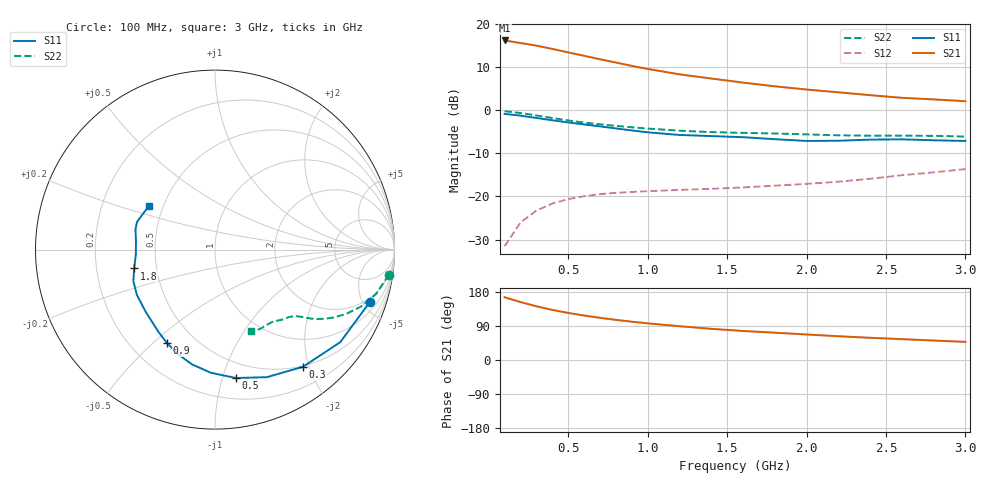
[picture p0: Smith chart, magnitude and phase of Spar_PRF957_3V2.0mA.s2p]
! Filename:  PRF957C.S2P  Version:  3.0
! NXP part #:  PRF957  Date:  Nov 1998
! Bias condition:  Vce=3V, Ic=2mA
#  MHz  S  MA  R 50
! Freq  S11  S21  S12  S22
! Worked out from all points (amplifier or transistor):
!   20 points, 100 MHz to 3 GHz, reference 50 ohm
!   highest |S21| = 16.2 dB at 100 MHz (marker M1)
!   |S21| within 3 dB of that: start of sweep to 528.3 MHz
!   unconditionally stable (mu >= 1): 1.815 GHz to end of sweep
!   at 400 MHz: K = 0.24, MSG = 18.0 dB, |S12| = -21.6 dB
!   at 1.2 GHz: K = 0.73, MSG = 13.4 dB, |S12| = -18.5 dB
!   at 3 GHz: K = 1.11, MAG = 5.9 dB, |S12| = -13.6 dB
!   S11 on the Smith chart (normalised r, x): 100 MHz: 1.63, -5.59; 300 MHz: 0.49, -1.90; 500 MHz: 0.37, -1.11; 900 MHz: 0.35, -0.55; 1.8 GHz: 0.37, -0.10; 3 GHz: 0.42, +0.25
100  0.9102 -18.8  6.486 165.5  0.02647 79.1  0.9783 -8.2
200  0.868 -36.4  6.058 152.9  0.04979 69.9  0.931 -15.4
300  0.8163 -53.1  5.648 141.8  0.06858 62.3  0.8732 -21.3
400  0.7672 -67.9  5.176 132.2  0.08272 56.3  0.8149 -26.0
500  0.7246 -80.8  4.711 124.2  0.0931 52.0  0.7638 -29.7
600  0.6868 -91.9  4.304 117.3  0.1007 48.9  0.7218 -32.3
700  0.6519 -101.4  3.925 111.3  0.1063 46.7  0.6883 -34.2
800  0.6171 -109.7  3.595 105.9  0.1101 45.3  0.6603 -35.6
900  0.5847 -117.3  3.287 101.1  0.1129 44.6  0.6362 -36.7
1000  0.556 -124.6  3.029 96.8  0.1152 44.5  0.615 -37.6
1200  0.5182 -138.4  2.623 89.1  0.1191 45.1  0.5805 -39.6
1400  0.503 -150.0  2.344 82.3  0.1227 46.7  0.5591 -42.2
1600  0.4881 -158.7  2.102 76.6  0.1272 49.8  0.5479 -44.6
1800  0.4626 -166.9  1.903 72.1  0.1334 53.5  0.5386 -46.6
2000  0.4416 -176.8  1.746 67.3  0.14 57.2  0.5259 -48.8
2200  0.4436 173.2  1.62 62.7  0.1484 60.8  0.5133 -52.0
2400  0.4573 165.8  1.502 58.6  0.1604 64.1  0.5078 -56.0
2600  0.4609 160.4  1.399 55.0  0.1766 67.0  0.5088 -59.5
2800  0.4494 154.6  1.341 51.3  0.1907 69.8  0.5058 -62.4
3000  0.4414 146.5  1.278 47.9  0.2079 72.1  0.4964 -65.8
